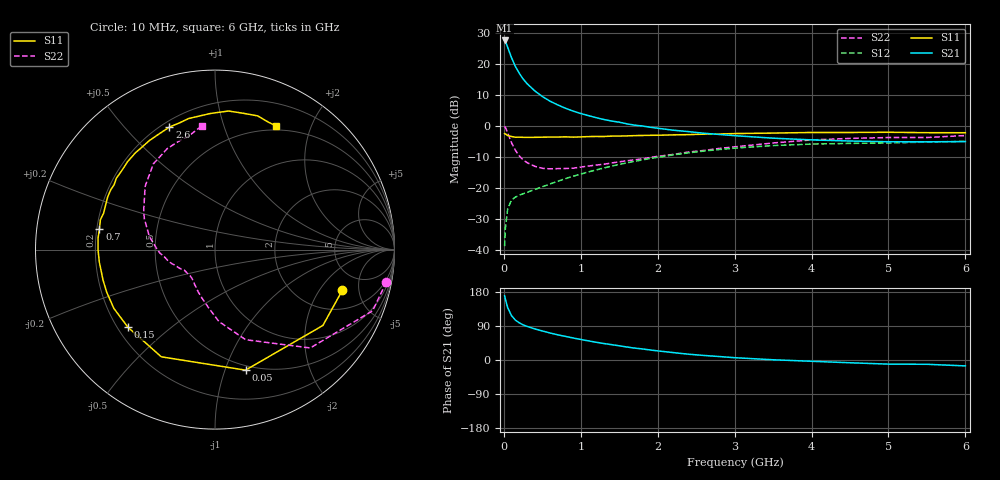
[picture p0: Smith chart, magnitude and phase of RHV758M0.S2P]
! SIEMENS Small Signal Semiconductors
! BFR106
! Si NPN RF Bipolar Junction Transistor in SOT23
! VCE = 0.75 V  IC = 8 mA
! Common Emitter S-Parameters:  August  1996
# GHz  S  MA  R  50
!  f  S11  S21  S12  S22
! GHz  MAG  ANG  MAG  ANG  MAG  ANG  MAG  ANG
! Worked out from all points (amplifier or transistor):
!   36 points, 10 MHz to 6 GHz, reference 50 ohm
!   highest |S21| = 27.5 dB at 10 MHz (marker M1)
!   |S21| within 3 dB of that: start of sweep to 61.72 MHz
!   unconditionally stable (mu >= 1): 489.4 MHz to end of sweep
!   at 250 MHz: K = 0.67, MSG = 18.5 dB, |S12| = -22.0 dB
!   at 1.4 GHz: K = 1.15, MAG = 5.0 dB, |S12| = -13.1 dB
!   at 6 GHz: K = 1.03, MAG = -1.1 dB, |S12| = -5.1 dB
!   S11 on the Smith chart (normalised r, x): 10 MHz: 3.30, -3.34; 50 MHz: 0.46, -1.18; 150 MHz: 0.24, -0.36; 700 MHz: 0.21, +0.09; 2.6 GHz: 0.23, +0.67; 6 GHz: 0.45, +1.52
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0.01  0.7451 -17.6  23.62 169.6  0.0114 82.5  0.9717 -10.7
0.02  0.7349 -35.1  22.88 160.6  0.0222 73.4  0.9422 -21.2
0.05  0.6928 -75.8  18.31 138.0  0.0457 55.8  0.7631 -45.9
0.1  0.668 -116.6  12.42 117.0  0.0633 41.8  0.5305 -71.2
0.15  0.6499 -138.2  8.991 105.3  0.0705 36.9  0.4018 -86.8
0.2  0.6518 -149.9  7.003 98.2  0.0754 36.4  0.3267 -96.2
0.25  0.6483 -158.5  5.664 92.7  0.0797 36.9  0.2798 -105.0
0.3  0.6466 -164.7  4.776 88.8  0.0839 38.4  0.2544 -111.4
0.4  0.6482 -173.8  3.653 82.2  0.0932 41.5  0.2214 -121.6
0.5  0.6516 -179.9  2.948 76.6  0.1033 44.6  0.2053 -128.6
0.6  0.6547 174.4  2.484 71.3  0.1148 47.0  0.201 -133.8
0.7  0.6543 169.7  2.161 66.5  0.1265 49.0  0.2028 -138.7
0.9  0.653 161.8  1.717 58.1  0.1529 51.1  0.206 -146.6
1.1  0.6661 153.8  1.45 50.4  0.1793 51.7  0.2235 -152.3
1.3  0.668 147.3  1.256 43.5  0.2079 51.3  0.2387 -158.7
1.6  0.6835 137.9  1.068 34.3  0.2516 49.5  0.2715 -167.5
2.2  0.7092 121.0  0.845 19.6  0.3376 42.1  0.3432 174.5
2.6  0.7284 110.4  0.754 12.0  0.3892 35.8  0.398 162.3
3.5  0.7587 92.0  0.628 0.6  0.4772 20.9  0.5253 137.8
4.5  0.7758 78.0  0.565 -7.3  0.5175 5.8  0.6224 115.3
5.5  0.7701 67.5  0.549 -11.3  0.5427 -3.2  0.6439 104.2
6  0.7685 63.6  0.553 -15.6  0.5582 -9.7  0.6922 96.2
